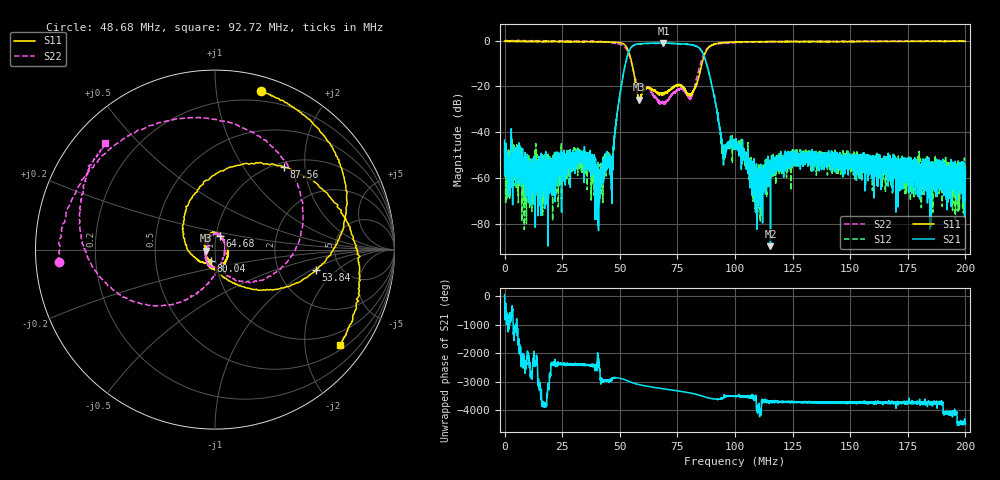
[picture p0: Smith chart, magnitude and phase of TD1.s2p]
#  HZ  S  DB  R  50.00
! Rohde & Schwarz Vector Network Analyzer
! Rohde-Schwarz,ZNL6-2Port,1323001206101378,1.50.1.34-21.10.1.104
! Created: UTC 7/31/2023, 2:26:56 AM
! freq[Hz]  db:S11  ang:S11  db:S21  ang:S21  db:S12  ang:S12  db:S22  ang:S22
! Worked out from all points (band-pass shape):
!   5001 points, 5 kHz to 200 MHz, reference 50 ohm
!   highest |S21| = -1.03 dB at 68.92 MHz (marker M1); lowest = -89.8 dB at 115.4 MHz (marker M2)
!   |S21| within 3 dB of the highest: 54.23 MHz to 85.24 MHz (31.02 MHz wide, 44.5 % of centre)
!   lowest |S11| = -25.8 dB at 58.48 MHz (marker M3), VSWR 1.11, Z = 45.2 - j0.476 ohm
!   |S11| at or under -10 dB: 55.28 MHz to 85.69 MHz (30.4 MHz wide, 43.1 % of centre)
!   |S22| runs from -27.8 to 0.1 dB; largest |S21 - S12| = 0.036
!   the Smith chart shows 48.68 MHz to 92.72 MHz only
!   S11 on the Smith chart (normalised r, x): 48.68 MHz: 0.12, +1.33; 53.84 MHz: 3.29, -1.11; 64.68 MHz: 1.04, +0.16; 80.04 MHz: 0.94, -0.12; 87.56 MHz: 1.08, +1.56; 92.72 MHz: 0.63, -2.85
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5000  -0.22 -179.7  -43.48 53.1  -47.45 -159.2  0.04 0.1
1.128472e7  -0.43 168.7  -71.96 139.8  -53.35 96.8  -0.03 -14.7
3.336417e7  -0.43 137.0  -50.83 139.3  -55.39 97.0  -0.12 -60.2
4.080398e7  -0.46 116.8  -62.08 -51.3  -63.15 -11.7  -0.36 -92.6
4.652384e7  -0.65 89.7  -52.49 -25.1  -54.09 -26.5  -0.79 -142.2
4.868378e7  -0.72 73.7  -33.16 22.1  -33.11 21.3  -1.20 -175.3
5.168371e7  -1.39 35.8  -13.86 -32.0  -13.85 -31.8  -2.39 107.2
5.384365e7  -4.82 -11.3  -4.91 -100.1  -5.02 -100.4  -5.73 18.2
5.848354e7  -25.85 -174.1  -1.40 138.4  -1.50 139.0  -19.58 -67.0
6.468338e7  -21.84 70.8  -1.08 46.1  -1.18 46.2  -23.69 -147.6
6.668333e7  -23.00 51.0  -1.12 21.8  -1.13 21.1  -27.08 177.3
6.892328e7  -22.87 7.6  -1.03 -5.5  -1.19 -5.0  -27.26 151.7
7.508312e7  -19.40 -87.7  -1.31 -77.1  -1.35 -77.9  -21.76 99.9
8.0043e7  -23.23 -111.2  -1.64 -143.7  -1.69 -143.5  -24.34 13.5
8.756281e7  -4.44 50.2  -9.68 55.6  -9.79 54.9  -3.78 -164.9
9.272268e7  -1.15 -37.2  -34.08 -7.7  -33.51 -10.4  -1.38 136.0
1.000025e8  -0.58 -81.3  -44.30 93.8  -44.78 98.1  -0.82 101.2
1.101222e8  -0.40 -108.6  -60.14 -98.4  -62.51 117.8  -0.57 76.9
1.154021e8  -0.45 -116.8  -89.82 -70.7  -57.52 -77.5  -0.46 68.6
1.333617e8  -0.40 -134.4  -57.12 -113.7  -50.84 -113.9  -0.32 51.2
1.666808e8  -0.32 -150.1  -56.89 -129.7  -55.77 -157.9  -0.19 34.6
2e8  -0.33 -158.7  -59.32 -129.3  -55.11 -126.1  -0.15 25.4
